(* Logix 5000 AddOnInstructionDefinition export Banner_IOLM_Param_M_v5; software revision 33.00 *)

TYPE Banner_IOL_Port_v5 :   // UDT that has all of the data items necessary to communicate with a specific Port on a IO-Link Master
STRUCT
   Port_Controlled : INT;   // Each bit represents a port on an IO-Link Master. Set to 1 to tell AOI to control that port.
   Port_Activate : INT;   // Each bit represents a port on an IO-Link Master. When ON that port will process any commands in queue.
   Port_Read : INT;   // Each bit represents a port on an IO-Link Master. Used to determine when device AOI has requested a Read command.
   Port_Write : INT;   // Each bit represents a port on an IO-Link Master. Used to determine when device AOI has requested a Write command.
   Port_RW_Complete : INT;   // Each bit represents a port on an IO-Link Master. Tells device AOI that Read or Write request has been completed.
   Port_Device_Read : INT;
   Data_Transfer : SINT[250];   // Array to transfer data from IO-Master to device AOIs.
END_STRUCT
END_TYPE

TYPE Banner_IOLM_EL_v5 :   // Error Log for Messages to IOLM.
STRUCT
   RW : SINT;   // 0 = Read, 1 = Write.
   Port : SINT;   // Port number that generated error.
   Index : INT;   // IO-Link Index for generated error.
END_STRUCT
END_TYPE

TYPE Banner_IOLM_v5 :   // UDT to control IO-Link Masters.
STRUCT
   Message_Source_Data : SINT[260];
   Message_Destination_Data : SINT[260];
   Error_Log : Banner_IOLM_EL_v5[10];
   Error_Write_Retry : BOOL;
   Num_Error_MSGS : DINT;
   IO_Link_Master_Busy : BOOL;   // 0 = While waiting for a command, 1 = Processing command
   AOI_Reset : BOOL;
   Port_Data : Banner_IOL_Port_v5;   // All of the necessary data to work with the various ports of the IO-Link Master.
   Halt_Operation : BOOL;   // When parameter is 1 the AOI is halted as next available time frame.
   AOI_Halted : BOOL;   // AOI is in standby mode until Halt Operation tag is set back to 0.
END_STRUCT
END_TYPE

ADD_ON_INSTRUCTION Banner_IOLM_Param_M_v5   (* revision 5.0, vendor Banner Engineering *)
// AOI that controls an Murr IO-Link Master with Banner devices for parameter data operations.
VAR_IN_OUT
   Message_Read : MESSAGE; {required}   // Message used to gather data from a device plugged into an Allen Bradley IO-Link Master.
   Message_Write : MESSAGE; {required}   // Message used to send parameter updates to a device plugged into an Allen Bradley IO-Link Master.
   IOLM : Banner_IOLM_v5; {required}
END_VAR
VAR_INPUT
   Type : DINT; {required}   // 0 = CIP Class = 80, 1 = CIP Class = 83. See manual for more information on ISDU format.
   Port1 : BOOL; {required}
   Port2 : BOOL; {required}
   Port3 : BOOL; {required}
   Port4 : BOOL; {required}
   Port5 : BOOL; {required}
   Port6 : BOOL; {required}
   Port7 : BOOL; {required}
   Port8 : BOOL; {required}
END_VAR
VAR_OUTPUT
   Done : BOOL; {visible}
   Busy : BOOL; {visible}
   Error : BOOL; {visible}
END_VAR
VAR
   Lock : DINT; {access None}
   Disable_Timer : BOOL; {access None}
   Byte_Length : SINT; {access None}
   Current_Port : INT; {access None}   // Current port to communicate with via the IO-Link Master.
   Array_Index : DINT; {access None}
   Data_Index : DINT; {access None}
   Message_Timer : TIMER := (PRE := 100); {access None}
   Error_Index : DINT; {access None}
   Message_Timer2 : TIMER := (PRE := 5000); {access None}
   Temp_Index : INT; {access None}
   Timer8 : TIMER := (PRE := 3000); {access None}
   WriteCnt : DINT; {access None}
   Last_Index : DINT; {access None}
   WrCntTotal : DINT; {access None}
END_VAR

ROUTINE Logic   (* ladder *)
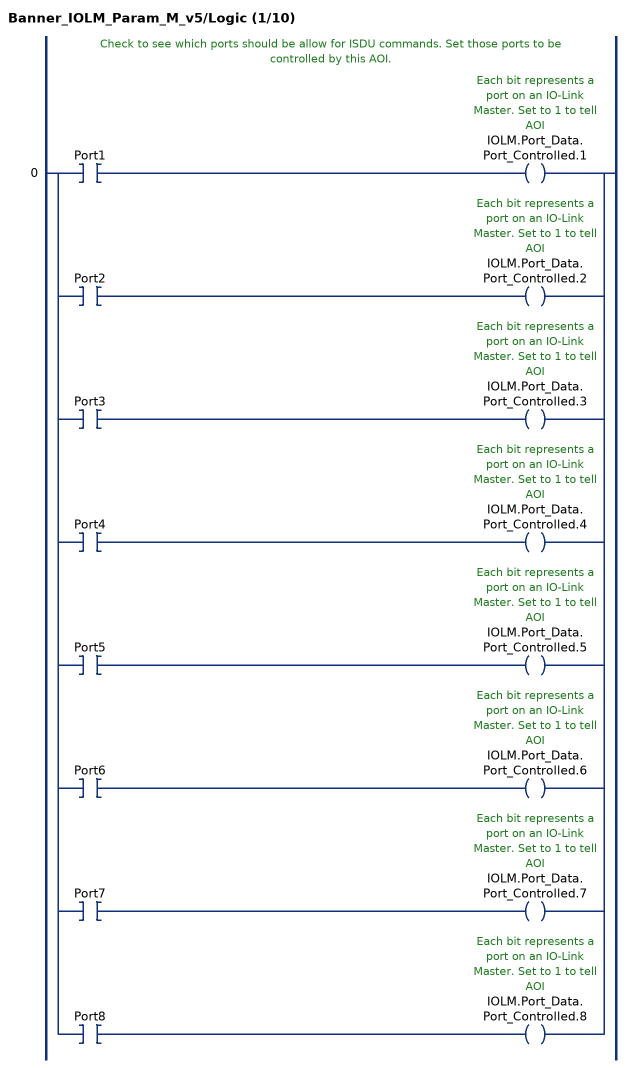
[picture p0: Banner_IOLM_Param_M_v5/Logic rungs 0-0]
   // Check to see which ports should be allow for ISDU commands. Set those ports to be controlled by this AOI.
   0: [XIC(Port1) OTE(IOLM.Port_Data.Port_Controlled.1) ,XIC(Port2) OTE(IOLM.Port_Data.Port_Controlled.2) ,XIC(Port3) OTE(IOLM.Port_Data.Port_Controlled.3) ,XIC(Port4) OTE(IOLM.Port_Data.Port_Controlled.4) ,XIC(Port5) OTE(IOLM.Port_Data.Port_Controlled.5) ,XIC(Port6) OTE(IOLM.Port_Data.Port_Controlled.6) ,XIC(Port7) OTE(IOLM.Port_Data.Port_Controlled.7) ,XIC(Port8) OTE(IOLM.Port_Data.Port_Controlled.8) ];
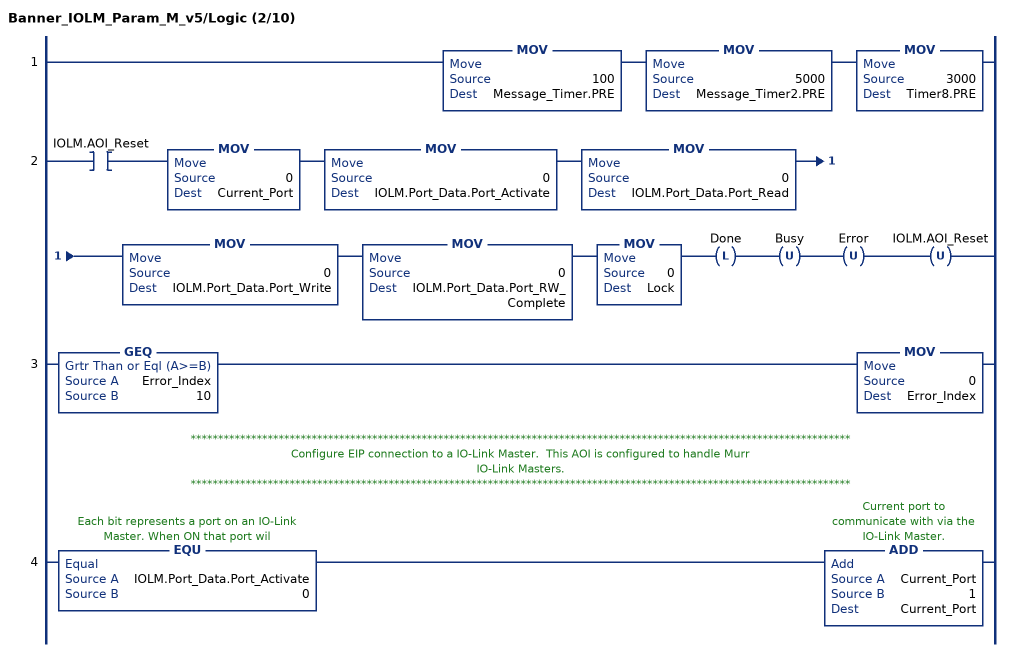
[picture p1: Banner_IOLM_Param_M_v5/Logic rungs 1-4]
   1: MOV(100,Message_Timer.PRE)MOV(5000,Message_Timer2.PRE)MOV(3000,Timer8.PRE);
   2: XIC(IOLM.AOI_Reset)MOV(0,Current_Port)MOV(0,IOLM.Port_Data.Port_Activate)MOV(0,IOLM.Port_Data.Port_Read)MOV(0,IOLM.Port_Data.Port_Write)MOV(0,IOLM.Port_Data.Port_RW_Complete)MOV(0,Lock)OTL(Done)OTU(Busy)OTU(Error)OTU(IOLM.AOI_Reset);
   3: GEQ(Error_Index,10)MOV(0,Error_Index);
   // ************************************************************************************************************************
   // Configure EIP connection to a IO-Link Master.  This AOI is configured to handle Murr
   // IO-Link Masters.
   // ************************************************************************************************************************
   4: EQU(IOLM.Port_Data.Port_Activate,0)ADD(Current_Port,1,Current_Port);
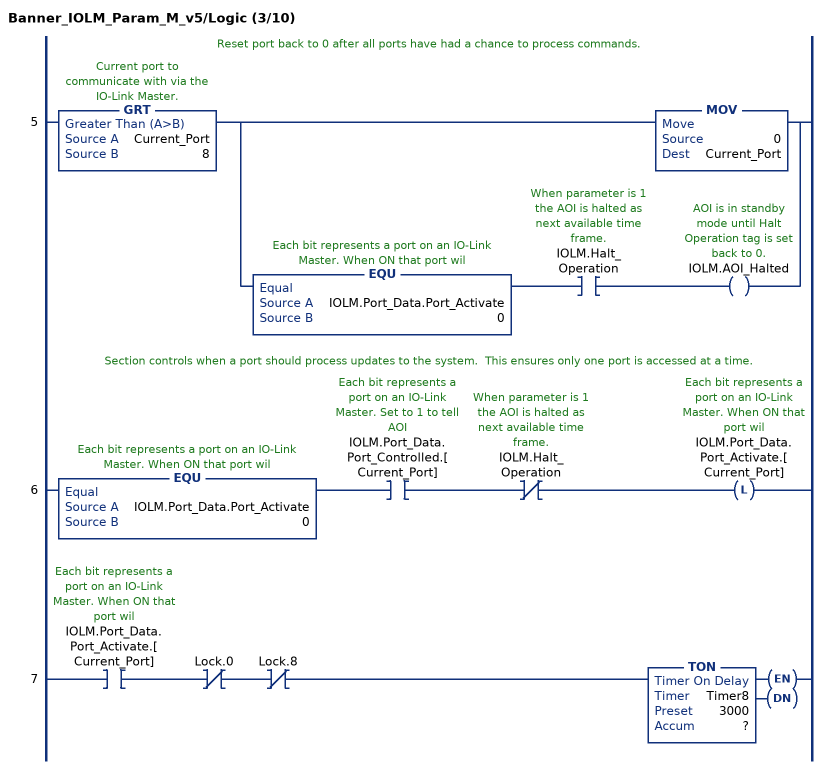
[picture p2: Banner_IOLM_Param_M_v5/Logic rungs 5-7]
   // Reset port back to 0 after all ports have had a chance to process commands.
   5: GRT(Current_Port,8)[MOV(0,Current_Port) ,EQU(IOLM.Port_Data.Port_Activate,0) XIC(IOLM.Halt_Operation) OTE(IOLM.AOI_Halted) ];
   // Section controls when a port should process updates to the system.  This ensures only one port is accessed at a time.
   6: EQU(IOLM.Port_Data.Port_Activate,0)XIC(IOLM.Port_Data.Port_Controlled.[Current_Port])XIO(IOLM.Halt_Operation)OTL(IOLM.Port_Data.Port_Activate.[Current_Port]);
   7: XIC(IOLM.Port_Data.Port_Activate.[Current_Port])XIO(Lock.0)XIO(Lock.8)TON(Timer8,?,?);
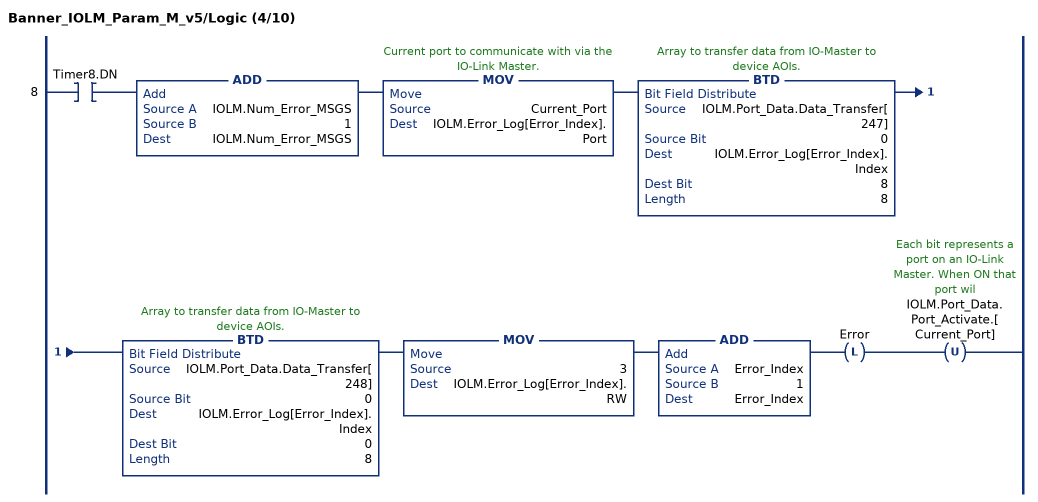
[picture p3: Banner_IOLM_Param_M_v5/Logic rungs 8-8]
   8: XIC(Timer8.DN)ADD(IOLM.Num_Error_MSGS,1,IOLM.Num_Error_MSGS)MOV(Current_Port,IOLM.Error_Log[Error_Index].Port)BTD(IOLM.Port_Data.Data_Transfer[247],0,IOLM.Error_Log[Error_Index].Index,8,8)BTD(IOLM.Port_Data.Data_Transfer[248],0,IOLM.Error_Log[Error_Index].Index,0,8)MOV(3,IOLM.Error_Log[Error_Index].RW)ADD(Error_Index,1,Error_Index)OTL(Error)OTU(IOLM.Port_Data.Port_Activate.[Current_Port]);
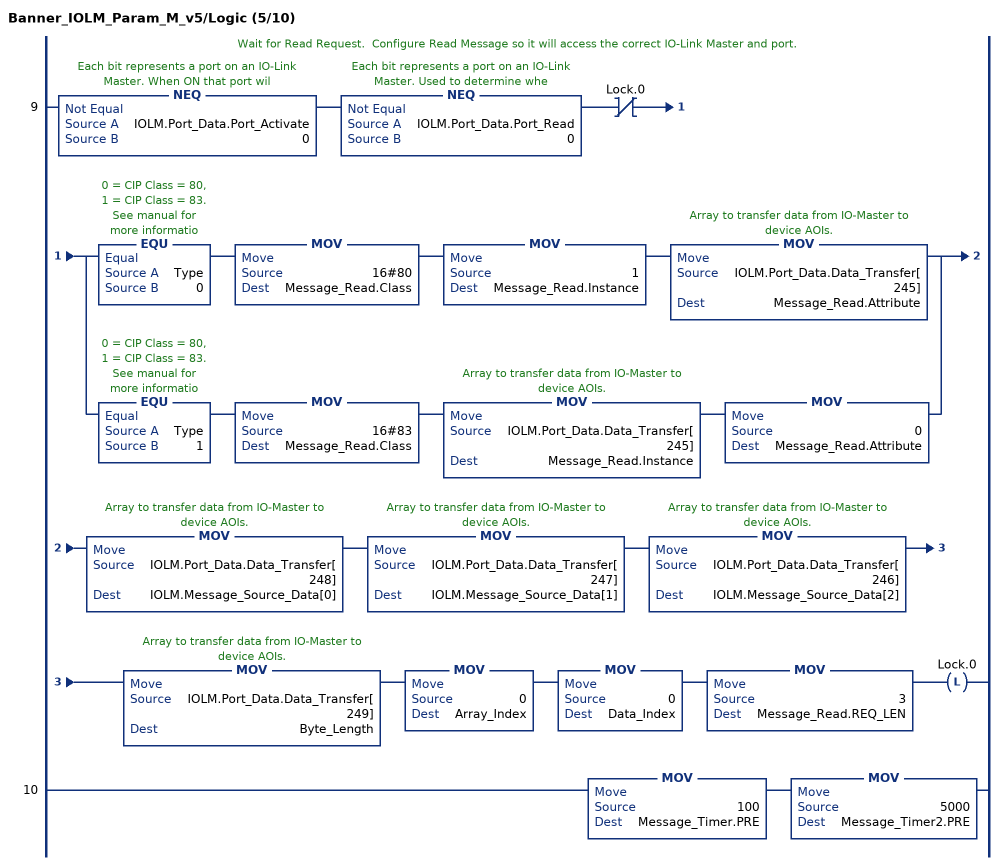
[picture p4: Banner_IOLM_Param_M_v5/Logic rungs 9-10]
   // Wait for Read Request.  Configure Read Message so it will access the correct IO-Link Master and port.
   9: NEQ(IOLM.Port_Data.Port_Activate,0)NEQ(IOLM.Port_Data.Port_Read,0)XIO(Lock.0)[EQU(Type,0) MOV(16#80,Message_Read.Class) MOV(1,Message_Read.Instance) MOV(IOLM.Port_Data.Data_Transfer[245],Message_Read.Attribute) ,EQU(Type,1) MOV(16#83,Message_Read.Class) MOV(IOLM.Port_Data.Data_Transfer[245],Message_Read.Instance) MOV(0,Message_Read.Attribute) ]MOV(IOLM.Port_Data.Data_Transfer[248],IOLM.Message_Source_Data[0])MOV(IOLM.Port_Data.Data_Transfer[247],IOLM.Message_Source_Data[1])MOV(IOLM.Port_Data.Data_Transfer[246],IOLM.Message_Source_Data[2])MOV(IOLM.Port_Data.Data_Transfer[249],Byte_Length)MOV(0,Array_Index)MOV(0,Data_Index)MOV(3,Message_Read.REQ_LEN)OTL(Lock.0);
   10: MOV(100,Message_Timer.PRE)MOV(5000,Message_Timer2.PRE);
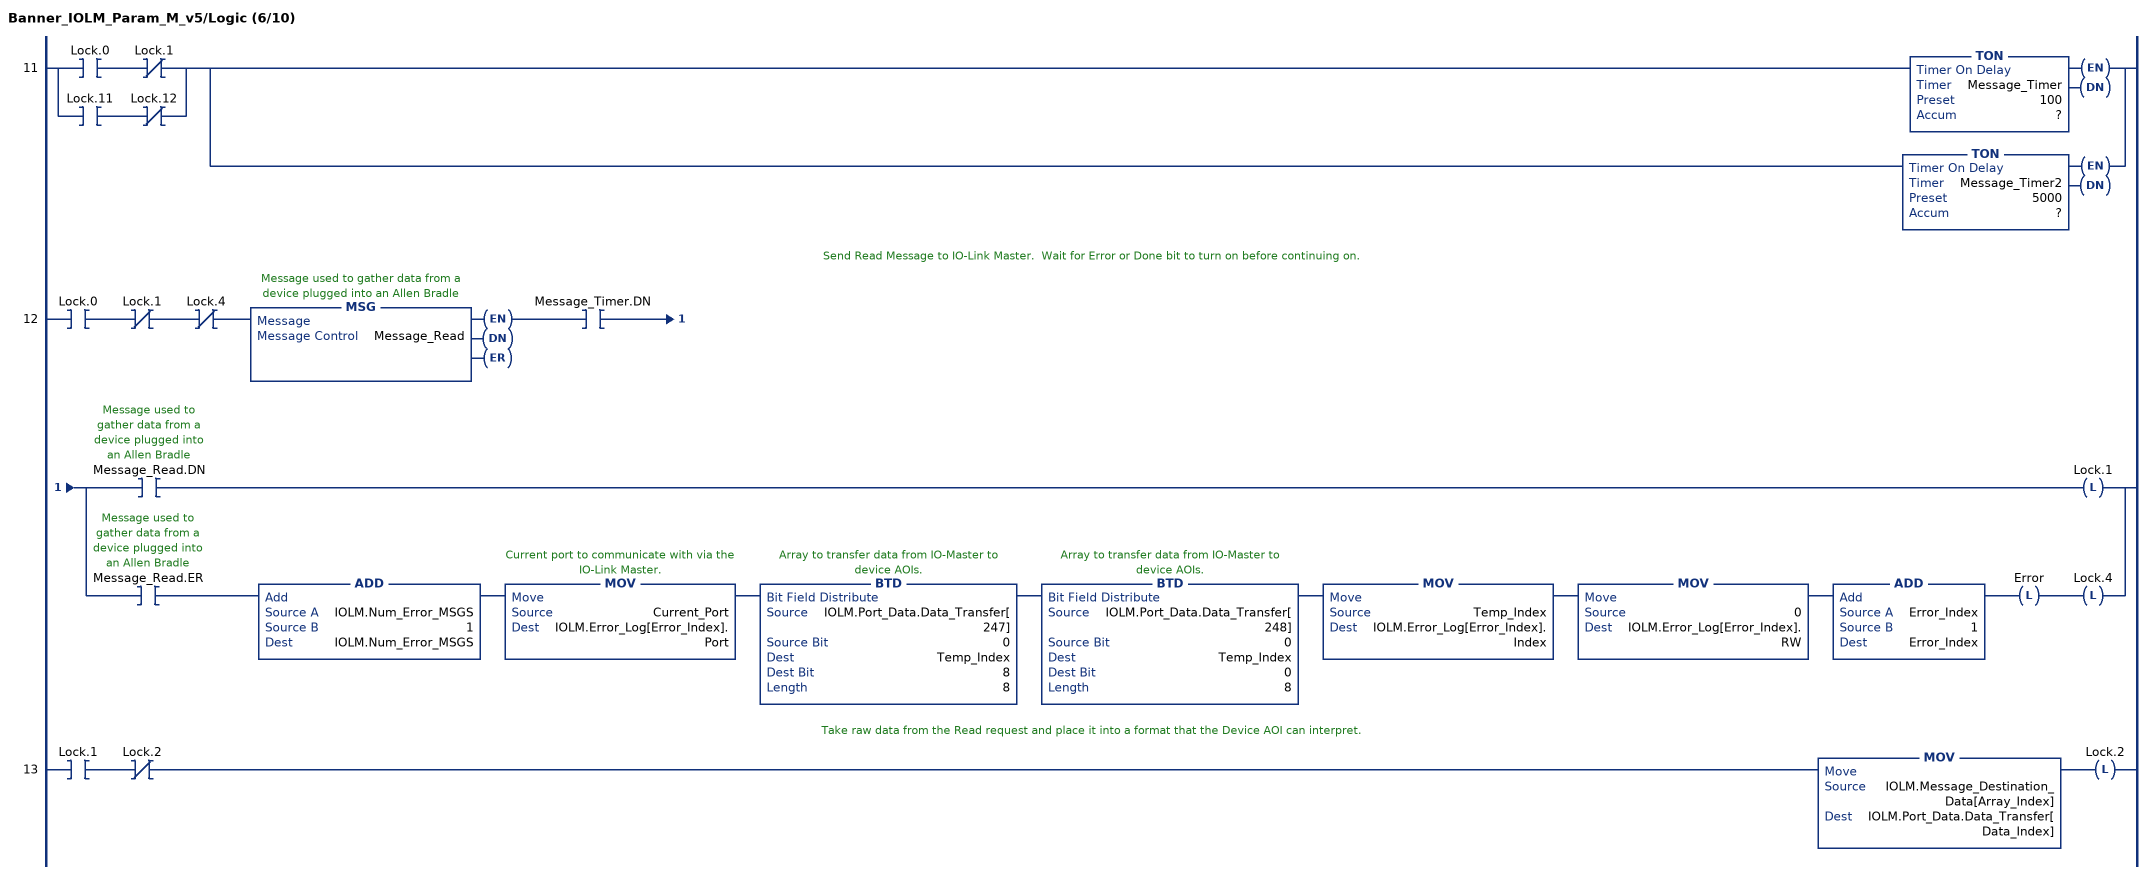
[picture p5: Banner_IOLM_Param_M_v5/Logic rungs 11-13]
   11: [XIC(Lock.0) XIO(Lock.1) ,XIC(Lock.11) XIO(Lock.12) ][TON(Message_Timer,?,?) ,TON(Message_Timer2,?,?) ];
   // Send Read Message to IO-Link Master.  Wait for Error or Done bit to turn on before continuing on.
   12: XIC(Lock.0)XIO(Lock.1)XIO(Lock.4)MSG(Message_Read)XIC(Message_Timer.DN)[XIC(Message_Read.DN) OTL(Lock.1) ,XIC(Message_Read.ER) ADD(IOLM.Num_Error_MSGS,1,IOLM.Num_Error_MSGS) MOV(Current_Port,IOLM.Error_Log[Error_Index].Port) BTD(IOLM.Port_Data.Data_Transfer[247],0,Temp_Index,8,8) BTD(IOLM.Port_Data.Data_Transfer[248],0,Temp_Index,0,8) MOV(Temp_Index,IOLM.Error_Log[Error_Index].Index) MOV(0,IOLM.Error_Log[Error_Index].RW) ADD(Error_Index,1,Error_Index) OTL(Error) OTL(Lock.4) ];
   // Take raw data from the Read request and place it into a format that the Device AOI can interpret.
   13: XIC(Lock.1)XIO(Lock.2)MOV(IOLM.Message_Destination_Data[Array_Index],IOLM.Port_Data.Data_Transfer[Data_Index])OTL(Lock.2);
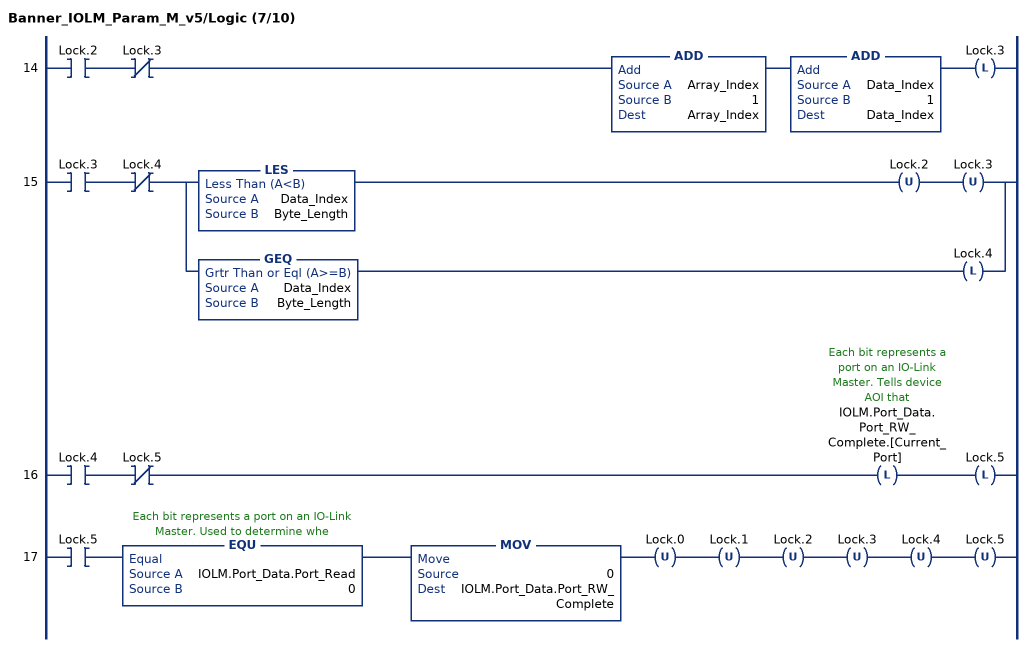
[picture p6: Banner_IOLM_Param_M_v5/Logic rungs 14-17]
   14: XIC(Lock.2)XIO(Lock.3)ADD(Array_Index,1,Array_Index)ADD(Data_Index,1,Data_Index)OTL(Lock.3);
   15: XIC(Lock.3)XIO(Lock.4)[LES(Data_Index,Byte_Length) OTU(Lock.2) OTU(Lock.3) ,GEQ(Data_Index,Byte_Length) OTL(Lock.4) ];
   16: XIC(Lock.4)XIO(Lock.5)OTL(IOLM.Port_Data.Port_RW_Complete.[Current_Port])OTL(Lock.5);
   17: XIC(Lock.5)EQU(IOLM.Port_Data.Port_Read,0)MOV(0,IOLM.Port_Data.Port_RW_Complete)OTU(Lock.0)OTU(Lock.1)OTU(Lock.2)OTU(Lock.3)OTU(Lock.4)OTU(Lock.5);
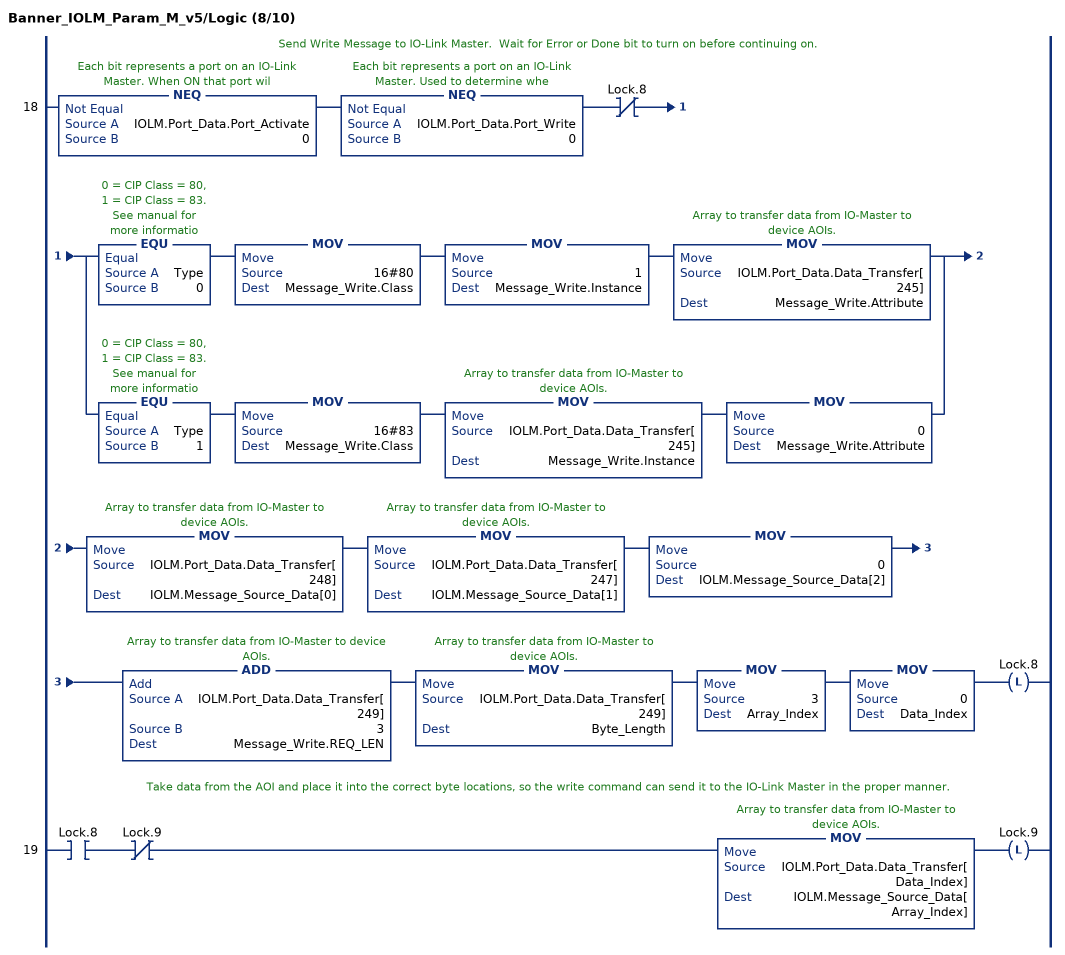
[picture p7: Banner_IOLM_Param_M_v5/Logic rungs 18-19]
   // Send Write Message to IO-Link Master.  Wait for Error or Done bit to turn on before continuing on.
   18: NEQ(IOLM.Port_Data.Port_Activate,0)NEQ(IOLM.Port_Data.Port_Write,0)XIO(Lock.8)[EQU(Type,0) MOV(16#80,Message_Write.Class) MOV(1,Message_Write.Instance) MOV(IOLM.Port_Data.Data_Transfer[245],Message_Write.Attribute) ,EQU(Type,1) MOV(16#83,Message_Write.Class) MOV(IOLM.Port_Data.Data_Transfer[245],Message_Write.Instance) MOV(0,Message_Write.Attribute) ]MOV(IOLM.Port_Data.Data_Transfer[248],IOLM.Message_Source_Data[0])MOV(IOLM.Port_Data.Data_Transfer[247],IOLM.Message_Source_Data[1])MOV(0,IOLM.Message_Source_Data[2])ADD(IOLM.Port_Data.Data_Transfer[249],3,Message_Write.REQ_LEN)MOV(IOLM.Port_Data.Data_Transfer[249],Byte_Length)MOV(3,Array_Index)MOV(0,Data_Index)OTL(Lock.8);
   // Take data from the AOI and place it into the correct byte locations, so the write command can send it to the IO-Link Master in the proper manner.
   19: XIC(Lock.8)XIO(Lock.9)MOV(IOLM.Port_Data.Data_Transfer[Data_Index],IOLM.Message_Source_Data[Array_Index])OTL(Lock.9);
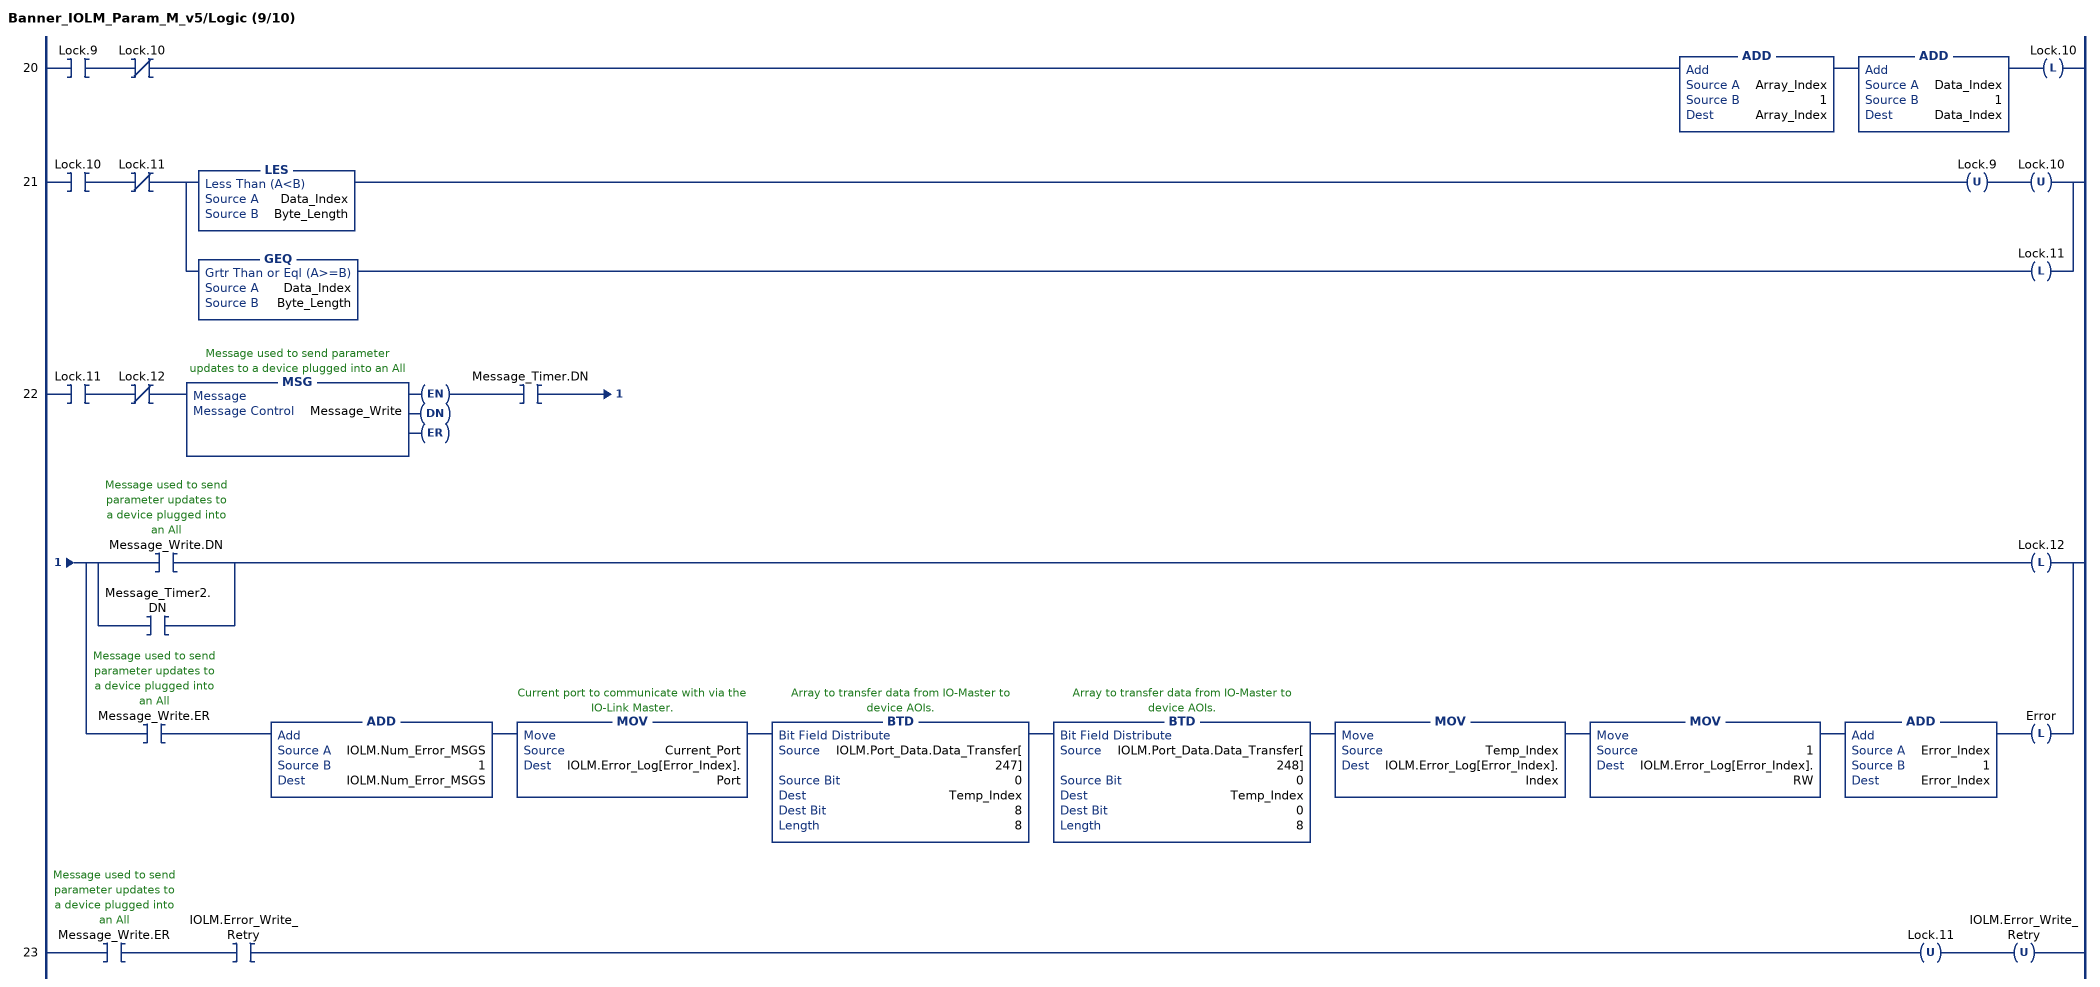
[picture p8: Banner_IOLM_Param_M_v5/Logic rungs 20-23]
   20: XIC(Lock.9)XIO(Lock.10)ADD(Array_Index,1,Array_Index)ADD(Data_Index,1,Data_Index)OTL(Lock.10);
   21: XIC(Lock.10)XIO(Lock.11)[LES(Data_Index,Byte_Length) OTU(Lock.9) OTU(Lock.10) ,GEQ(Data_Index,Byte_Length) OTL(Lock.11) ];
   22: XIC(Lock.11)XIO(Lock.12)MSG(Message_Write)XIC(Message_Timer.DN)[[XIC(Message_Write.DN) ,XIC(Message_Timer2.DN) ] OTL(Lock.12) ,XIC(Message_Write.ER) ADD(IOLM.Num_Error_MSGS,1,IOLM.Num_Error_MSGS) MOV(Current_Port,IOLM.Error_Log[Error_Index].Port) BTD(IOLM.Port_Data.Data_Transfer[247],0,Temp_Index,8,8) BTD(IOLM.Port_Data.Data_Transfer[248],0,Temp_Index,0,8) MOV(Temp_Index,IOLM.Error_Log[Error_Index].Index) MOV(1,IOLM.Error_Log[Error_Index].RW) ADD(Error_Index,1,Error_Index) OTL(Error) ];
   23: XIC(Message_Write.ER)XIC(IOLM.Error_Write_Retry)OTU(Lock.11)OTU(IOLM.Error_Write_Retry);
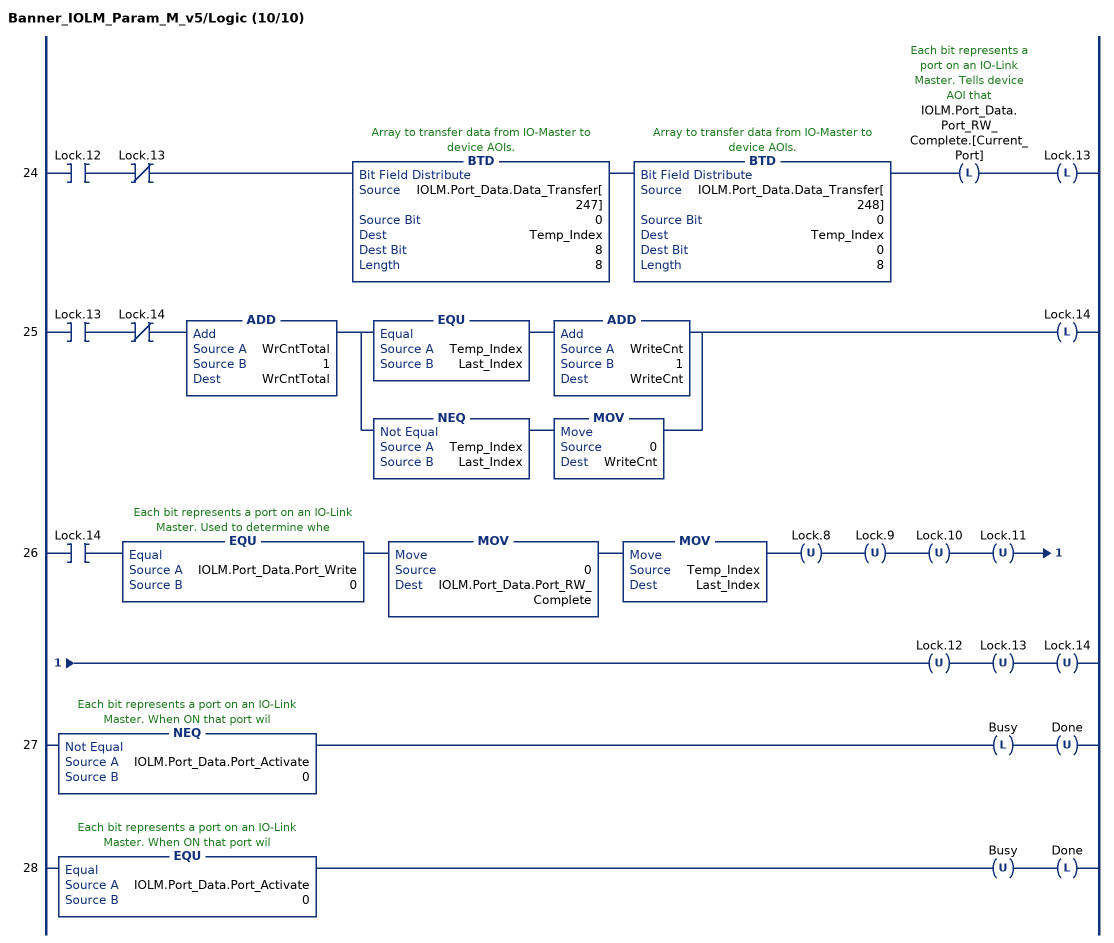
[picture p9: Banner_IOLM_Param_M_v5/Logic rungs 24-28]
   24: XIC(Lock.12)XIO(Lock.13)BTD(IOLM.Port_Data.Data_Transfer[247],0,Temp_Index,8,8)BTD(IOLM.Port_Data.Data_Transfer[248],0,Temp_Index,0,8)OTL(IOLM.Port_Data.Port_RW_Complete.[Current_Port])OTL(Lock.13);
   25: XIC(Lock.13)XIO(Lock.14)ADD(WrCntTotal,1,WrCntTotal)[EQU(Temp_Index,Last_Index) ADD(WriteCnt,1,WriteCnt) ,NEQ(Temp_Index,Last_Index) MOV(0,WriteCnt) ]OTL(Lock.14);
   26: XIC(Lock.14)EQU(IOLM.Port_Data.Port_Write,0)MOV(0,IOLM.Port_Data.Port_RW_Complete)MOV(Temp_Index,Last_Index)OTU(Lock.8)OTU(Lock.9)OTU(Lock.10)OTU(Lock.11)OTU(Lock.12)OTU(Lock.13)OTU(Lock.14);
   27: NEQ(IOLM.Port_Data.Port_Activate,0)OTL(Busy)OTU(Done);
   28: EQU(IOLM.Port_Data.Port_Activate,0)OTU(Busy)OTL(Done);
END_ROUTINE
END_ADD_ON_INSTRUCTION
